(* Logix 5000 AddOnInstructionDefinition export FRA7NWIE_Generic_Default_IO; software revision 19.01 *)

ADD_ON_INSTRUCTION FRA7NWIE_Generic_Default_IO   (* revision 1.0 *)
// Simple interface for generic default IO mapping that uses Input Assembly Instance 150 and Output Assembly Instance 100.
VAR_IN_OUT
   I_Data : INT[2]; {required}   // Input data
   O_Data : INT[2]; {required}   // Output data
END_VAR
VAR_INPUT
   RunStop : BOOL; {access Read Only, required}   // Run (0) or Stop (1)
   Forward : BOOL; {access Read Only, required}   // Run forward direction
   Reverse : BOOL; {required}   // Run reverse direction
   Reset : BOOL; {required}   // Reset the fault
   FrequencyCommand : INT; {access Read Only, required}   // Frequency command/reference
END_VAR
VAR_OUTPUT
   RunningStopped : BOOL; {access Read Only, visible}   // Running (1) or Stopped (0)
   RunningForward : BOOL; {visible}   // Running forward direction
   RunningReverse : BOOL; {visible}   // Running reverse direction
   UpToFrequency : BOOL; {access Read Only, visible}   // Up to frequency
   Alarm : BOOL; {access Read Only, visible}   // Alarm or Trip
   OutputFrequency : INT; {access Read Only, visible}   // Output/feedback frequency
END_VAR

ROUTINE Logic   (* ladder *)
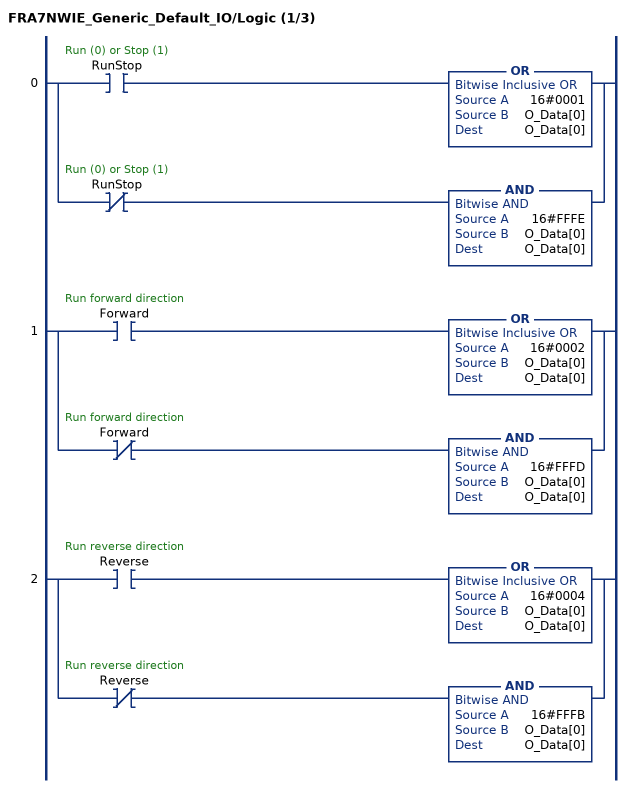
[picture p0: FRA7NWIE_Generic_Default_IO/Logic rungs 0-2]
   0: [XIC(RunStop) OR(16#0001,O_Data[0],O_Data[0]) ,XIO(RunStop) AND(16#FFFE,O_Data[0],O_Data[0]) ];
   1: [XIC(Forward) OR(16#0002,O_Data[0],O_Data[0]) ,XIO(Forward) AND(16#FFFD,O_Data[0],O_Data[0]) ];
   2: [XIC(Reverse) OR(16#0004,O_Data[0],O_Data[0]) ,XIO(Reverse) AND(16#FFFB,O_Data[0],O_Data[0]) ];
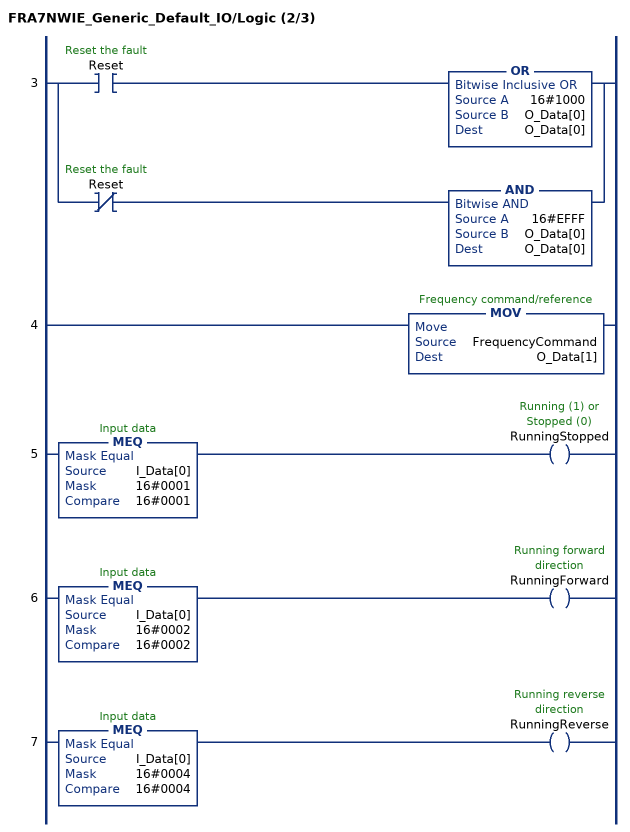
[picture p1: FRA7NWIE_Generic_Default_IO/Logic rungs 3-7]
   3: [XIC(Reset) OR(16#1000,O_Data[0],O_Data[0]) ,XIO(Reset) AND(16#EFFF,O_Data[0],O_Data[0]) ];
   4: MOV(FrequencyCommand,O_Data[1]);
   5: MEQ(I_Data[0],16#0001,16#0001)OTE(RunningStopped);
   6: MEQ(I_Data[0],16#0002,16#0002)OTE(RunningForward);
   7: MEQ(I_Data[0],16#0004,16#0004)OTE(RunningReverse);
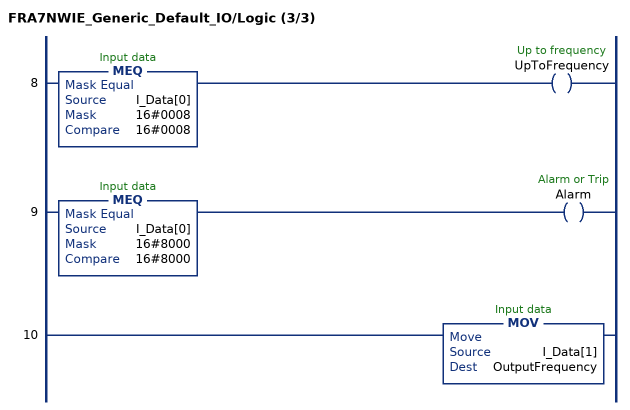
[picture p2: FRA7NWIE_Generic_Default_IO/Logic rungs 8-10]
   8: MEQ(I_Data[0],16#0008,16#0008)OTE(UpToFrequency);
   9: MEQ(I_Data[0],16#8000,16#8000)OTE(Alarm);
   10: MOV(I_Data[1],OutputFrequency);
END_ROUTINE
END_ADD_ON_INSTRUCTION
